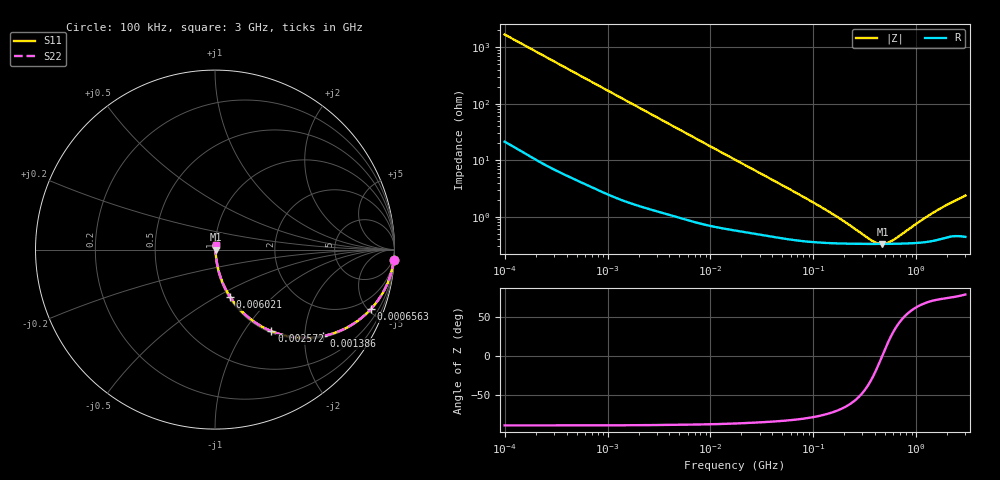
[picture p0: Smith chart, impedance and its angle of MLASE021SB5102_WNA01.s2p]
! MLASE021SB5102_WNA01  S-PARAMETER MODEL  ( Standard Model )
! Model Generated by TAIYO YUDEN Corporation (http://www.ty-top.com)
! Version 1.0
! TAIYO YUDEN Control No. 220901
! Copyright(c) 2022 TAIYO YUDEN CO.,LTD. All Rights Reserved.
! Product Description (link to TY-COMPAS)
! https://ds.yuden.co.jp/TYCOMPAS/or/detail?pn=MLASE021SB5102KWNA01&u=M
! Products Name : Multilayer Ceramic Capacitors
! Characteristics :
!  Capacitance : 1000 [pF] , Rated Voltage : 16 [V] , TCC : X5R
!  Case Size : 0.25 x 0.125 / 0.0098 x 0.0049 [mm/inch] , Thickness : 0.125 / 0.0049 [mm/inch]
!  (Conditions: Temperature = 25 [degC] , DC Bias Voltage = 0 [V])
! External Node Assignments :
!  1  o---| |---o  2
! GND o---------o GND
! Frequency Range : 100kHz  -  3GHz  [ 401 STEP ]
# MHZ S RI R 50
! Freq[MHz].  S11 Real  S11 Imag  S21 Real  S21 Imag  S12 Real  S12 Imag  S22 Real  S22 Imag
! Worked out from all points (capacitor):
!   401 points, 100 kHz to 3 GHz, reference 50 ohm
!   read as one part in series: C = 943 pF near 105.3 kHz
!   lowest |Z| = 328 mohm at 469.1 MHz (marker M1)
!   series resonance near 465.8 MHz, so ESL is about 120 pH
!   S11 on the Smith chart (normalised r, x): 100 kHz: 1, -34; 656.3 kHz: 1.07, -5.21; 1.386 MHz: 1.04, -2.48; 2.572 MHz: 1.03, -1.34; 6.021 MHz: 1.02, -0.58; 3 GHz: 1.01, +0.05
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0.1  0.9958 -0.0591  0.00425 0.0591  0.00425 0.0591  0.9958 -0.0591
0.246461  0.9777 -0.1418  0.0223 0.1418  0.0223 0.1418  0.9777 -0.1418
0.562235  0.8989 -0.2949  0.1011 0.2949  0.1011 0.2949  0.8989 -0.2949
0.656258  0.8681 -0.3317  0.1319 0.3317  0.1319 0.3317  0.8681 -0.3317
0.941399  0.7648 -0.417  0.2352 0.417  0.2352 0.417  0.7648 -0.417
1.385689  0.6041 -0.4813  0.3959 0.4813  0.3959 0.4813  0.6041 -0.4813
1.887902  0.4547 -0.4892  0.5453 0.4892  0.5453 0.4892  0.4547 -0.4892
2.572132  0.3139 -0.4541  0.6861 0.4541  0.6861 0.4541  0.3139 -0.4541
3.161081  0.2352 -0.4132  0.7648 0.4132  0.7648 0.4132  0.2352 -0.4132
4.306746  0.1459 -0.3405  0.8541 0.3405  0.8541 0.3405  0.1459 -0.3405
6.020821  0.0839 -0.2627  0.9161 0.2627  0.9161 0.2627  0.0839 -0.2627
10.08119  0.0355 -0.1664  0.9645 0.1664  0.9645 0.1664  0.0355 -0.1664
17.7727  0.0152 -0.0972  0.9848 0.0972  0.9848 0.0972  0.0152 -0.0972
37.52708  0.00669 -0.047  0.9933 0.047  0.9933 0.047  0.00669 -0.047
97.38194  0.00385 -0.0178  0.9962 0.0178  0.9962 0.0178  0.00385 -0.0178
180.7614  0.0034 -0.00855  0.9966 0.00855  0.9966 0.00855  0.0034 -0.00855
362.5028  0.00327 -0.00198  0.9967 0.00198  0.9967 0.00198  0.00327 -0.00198
412.3589  0.00327 -0.000956  0.9967 0.000956  0.9967 0.000956  0.00327 -0.000956
469.0719  0.00327 5.58e-05  0.9967 -5.58e-05  0.9967 -5.58e-05  0.00327 5.58e-05
547.5153  0.00328 0.00127  0.9967 -0.00127  0.9967 -0.00127  0.00328 0.00127
1495.945  0.00386 0.0114  0.9961 -0.0114  0.9961 -0.0114  0.00386 0.0114
3000  0.00488 0.0229  0.9951 -0.0229  0.9951 -0.0229  0.00488 0.0229
